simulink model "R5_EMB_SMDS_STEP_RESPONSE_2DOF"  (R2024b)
settings: Solver=ode5  StartTime=0.0  StopTime=S  FixedStep=T  RelTol=1e-3  EnableMultiTasking=on
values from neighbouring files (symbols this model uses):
  Kt = 0.0273    [R5_EMB_SMDS_STEP_RESPONESE_2DOF_script.m]
  r_act = 0.0105    [R5_EMB_SMDS_STEP_RESPONESE_2DOF_script.m]
  T = 0.002    [R5_EMB_SMDS_STEP_RESPONESE_2DOF_script.m]
undefined symbols (not defined in the file or in its folder): Serial_Port, Standard_Devices
libraries: easyio x7, simulink x1

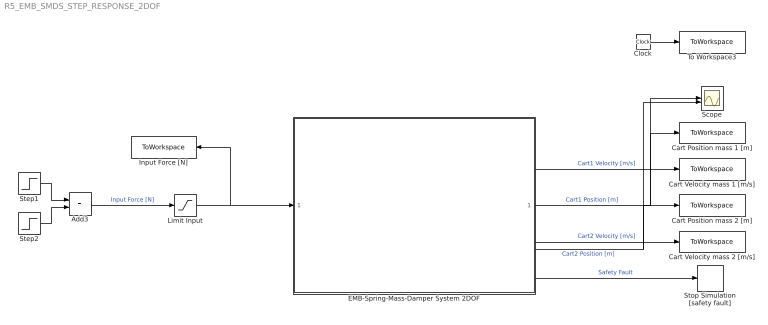
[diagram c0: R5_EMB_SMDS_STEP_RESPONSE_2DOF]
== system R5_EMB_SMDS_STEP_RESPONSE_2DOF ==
  Add3 : Sum
  Cart Position mass 1 [m] : ToWorkspace  VariableName=cart1_position  SampleTime=-1
  Cart Position mass 2 [m] : ToWorkspace  VariableName=cart2_position  SampleTime=-1
  Cart Velocity mass 1 [m/s] : ToWorkspace  VariableName=cart1_velocity  SampleTime=-1
  Cart Velocity mass 2 [m/s] : ToWorkspace  VariableName=cart2_velocity  SampleTime=-1
  Clock : Clock
  EMB-Spring-Mass-Damper System 2DOF : Subsystem
  Input Force [N] : ToWorkspace  VariableName=f_input  SampleTime=-1
  Limit Input : Saturate  UpperLimit=10  LowerLimit=-10
  Scope : Scope  NumInputPorts=2
  Step1 : Step  After=5  SampleTime=0
  Step2 : Step  Time=2  After=-5  SampleTime=0
  Stop Simulation [safety fault] : Stop
  To Workspace3 : ToWorkspace  VariableName=rt_time  SampleTime=-1
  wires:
  Clock/1 -> To Workspace3/1
  EMB-Spring-Mass-Damper System 2DOF/1(Out1) -> Scope/1, Cart Position mass 1 [m]/1  "Cart1 Position [m]"
  EMB-Spring-Mass-Damper System 2DOF/5(Out3) -> Stop Simulation [safety fault]/1  "Safety Fault"
  EMB-Spring-Mass-Damper System 2DOF/2(Out2) -> Cart Velocity mass 1 [m/s]/1  "Cart1 Velocity [m/s]"
  Step1/1 -> Add3/1
  Step2/1 -> Add3/2
  Limit Input/1 -> Input Force [N]/1, EMB-Spring-Mass-Damper System 2DOF/1(In1)
  EMB-Spring-Mass-Damper System 2DOF/3(Out4) -> Scope/2, Cart Position mass 2 [m]/1  "Cart2 Position [m]"
  EMB-Spring-Mass-Damper System 2DOF/4(Out5) -> Cart Velocity mass 2 [m/s]/1  "Cart2 Velocity [m/s]"
  Add3/1 -> Limit Input/1  "Input Force [N]"

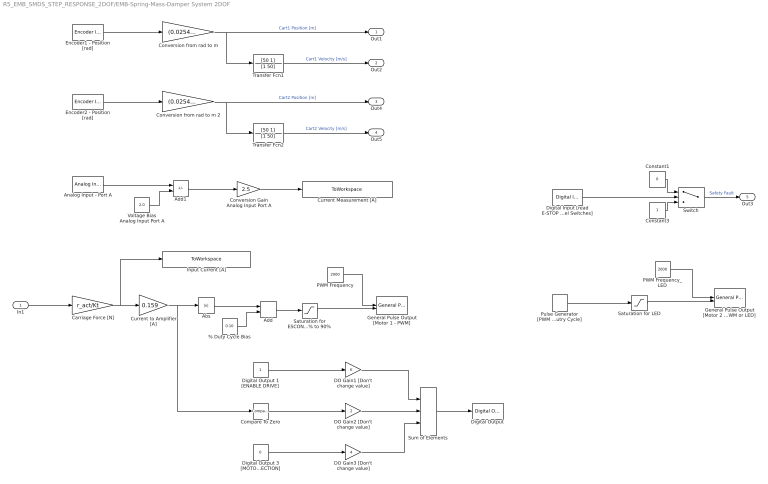
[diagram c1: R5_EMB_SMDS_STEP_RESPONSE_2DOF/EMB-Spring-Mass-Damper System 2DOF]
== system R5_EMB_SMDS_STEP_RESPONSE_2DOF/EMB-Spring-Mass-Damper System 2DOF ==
  In1 : Inport
  % Duty Cycle Bias : Constant  Value=0.10
  Abs : Abs
  Add : Sum
  Add1 : Sum  Inputs=+-
  Analog Input - Port A : easyio/Analog Input  SampleTime=T  MaxMissedTicks=10  ShowMissedTicks=0  YieldWhenWaiting=0  DrvName=Standard_Devices/Serial_Port  DrvAddress=6  DrvOptions=[460800 8 0 0 0 0 0 0]  PacketSize=8  DataTypes='double'  ShowReady=0  ShowError=0  PacketID=1  ByteOrder=1  ShowTimestamp=0  CfgPrm=A6  PrmCfg=unipolar  ResVar=0  VarRes=0
  Carriage Force [N] : Gain  Gain=r_act/Kt
  Compare To Zero : simulink/Logic and Bit Operations/Compare To Zero  relop=>=  OutDataTypeStr=boolean
  Constant1 : Constant  Value=0
  Constant3 : Constant
  Conversion Gain Analog Input Port A : Gain  Gain=2.5
  Conversion from rad to m : Gain  Gain=(0.0254)/(2*pi)
  Conversion from rad to m 2 : Gain  Gain=(0.0254)/(2*pi)
  Current Measurement [A] : ToWorkspace  VariableName=i_measure  SampleTime=-1
  Current to Amplifier [A] : Gain  Gain=0.159
  DO Gain1 [Don't change value] : Gain
  DO Gain2 [Don't change value] : Gain  Gain=2
  DO Gain3 [Don't change value] : Gain  Gain=4
  Digital Input [read E-STOP and End of Travel Switches] : easyio/Digital Input  SampleTime=T  MaxMissedTicks=10  ShowMissedTicks=0  YieldWhenWaiting=0  DrvName=Standard_Devices/Serial_Port  DrvAddress=6  DrvOptions=[460800 8 0 0 0 0 0 0]  PacketSize=8  DataTypes='double'  ShowReady=0  ShowError=0  PacketID=1  ByteOrder=1  ShowTimestamp=0  CfgPrm=D0  PrmCfg=18  ResVar=0  VarRes=0  d7=off  d6=off  d5=off  d4=on  d3=on  d2=off  d1=off  d0=off
  Digital Output : easyio/Digital Output  SampleTime=T  MaxMissedTicks=10  ShowMissedTicks=0  YieldWhenWaiting=0  DrvName=Standard_Devices/Serial_Port  DrvAddress=6  DrvOptions=[460800 8 0 0 0 0 0 0]  PacketSize=8  DataTypes='double'  ShowReady=0  ShowError=0  PacketID=1  ByteOrder=1  InitialValue=0  FinalValue=0  CfgPrm=G0  PrmCfg=F8  ResVar=0  VarRes=0  d7=off  d6=off  d5=off  d4=off  d3=off  d2=on  d1=on  d0=on
  Digital Output 1 [ENABLE DRIVE] : Constant
  Digital Output 3 [MOTOR 2 DIRECTION] : Constant  Value=0
  Encoder1 - Position [rad] : easyio/Encoder Input  SampleTime=T  MaxMissedTicks=10  ShowMissedTicks=0  YieldWhenWaiting=0  DrvName=Standard_Devices/Serial_Port  DrvAddress=6  DrvOptions=[460800 8 0 0 0 0 0 0]  PacketSize=8  DataTypes='double'  ShowReady=0  ShowError=0  PacketID=1  ByteOrder=1  ShowTimestamp=0  CfgPrm=E0  PrmCfg=position  ResVar=0  VarRes=2000
  Encoder2 - Position [rad] : easyio/Encoder Input  SampleTime=T  MaxMissedTicks=10  ShowMissedTicks=0  YieldWhenWaiting=0  DrvName=Standard_Devices/Serial_Port  DrvAddress=6  DrvOptions=[460800 8 0 0 0 0 0 0]  PacketSize=8  DataTypes='double'  ShowReady=0  ShowError=0  PacketID=1  ByteOrder=1  ShowTimestamp=0  CfgPrm=E1  PrmCfg=position  ResVar=0  VarRes=2000
  General Pulse Output [Motor 1 - PWM] : easyio/General Pulse Output  SampleTime=T  MaxMissedTicks=10  ShowMissedTicks=0  YieldWhenWaiting=0  DrvName=Standard_Devices/Serial_Port  DrvAddress=6  DrvOptions=[460800 8 0 0 0 0 0 0]  PacketSize=16  DataTypes={'double','double'}  ShowReady=0  ShowError=0  PacketID=1  ByteOrder=1  InitialValue=[0 0]  FinalValue=[0 0]  CfgPrm=N0  PrmCfg=frequency and duty  ResVar=449.8360 Hz - 115156.25 Hz  VarRes=64
  General Pulse Output [Motor 2 - PWM or LED] : easyio/General Pulse Output  SampleTime=T  MaxMissedTicks=10  ShowMissedTicks=0  YieldWhenWaiting=0  DrvName=Standard_Devices/Serial_Port  DrvAddress=6  DrvOptions=[460800 8 0 0 0 0 0 0]  PacketSize=16  DataTypes={'double','double'}  ShowReady=0  ShowError=0  PacketID=1  ByteOrder=1  InitialValue=[0 0]  FinalValue=[0 0]  CfgPrm=N1  PrmCfg=frequency and duty  ResVar=449.8360 Hz - 115156.25 Hz  VarRes=64
  Input Current [A] : ToWorkspace  VariableName=i_input  SampleTime=-1
  PWM Frequency : Constant  Value=2000
  PWM Frequency_LED : Constant  Value=2000
  Pulse Generator [PWM % Dutry Cycle] : DiscretePulseGenerator  PulseType=Time based  Period=0.4  PulseWidth=50
  Saturation for ESCON 10% to 90% : Saturate  UpperLimit=0.9  LowerLimit=0.1
  Saturation for LED : Saturate  UpperLimit=1  LowerLimit=0
  Sum of Elements : Sum  Inputs=+++
  Switch : Switch  Threshold=8
  Transfer Fcn1 : TransferFcn  Numerator=[50 1]  Denominator=[1 50]
  Transfer Fcn2 : TransferFcn  Numerator=[50 1]  Denominator=[1 50]
  Voltage Bias Analog Input Port A : Constant  Value=2.0
  Out1 : Outport
  Out2 : Outport  Port=2
  Out4 : Outport  Port=3
  Out5 : Outport  Port=4
  Out3 : Outport  Port=5
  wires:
  % Duty Cycle Bias/1 -> Add/2
  Conversion Gain Analog Input Port A/1 -> Current Measurement [A]/1
  Add1/1 -> Conversion Gain Analog Input Port A/1
  Constant1/1 -> Switch/1
  Current to Amplifier [A]/1 -> Abs/1, Compare To Zero/1
  Saturation for ESCON 10% to 90%/1 -> General Pulse Output [Motor 1 - PWM]/2
  Voltage Bias Analog Input Port A/1 -> Add1/2
  DO Gain2 [Don't change value]/1 -> Sum of Elements/2
  Analog Input - Port A/1 -> Add1/1
  PWM Frequency/1 -> General Pulse Output [Motor 1 - PWM]/1
  Conversion from rad to m/1 -> Out1/1, Transfer Fcn1/1  "Cart1 Position [m]"
  DO Gain1 [Don't change value]/1 -> Sum of Elements/1
  Digital Output 1 [ENABLE DRIVE]/1 -> DO Gain1 [Don't change value]/1
  Saturation for LED/1 -> General Pulse Output [Motor 2 - PWM or LED]/2
  Digital Input [read E-STOP and End of Travel Switches]/1 -> Switch/2
  PWM Frequency_LED/1 -> General Pulse Output [Motor 2 - PWM or LED]/1
  Carriage Force [N]/1 -> Input Current [A]/1, Current to Amplifier [A]/1
  Pulse Generator [PWM % Dutry Cycle]/1 -> Saturation for LED/1
  Encoder1 - Position [rad]/1 -> Conversion from rad to m/1
  Sum of Elements/1 -> Digital Output/1
  Add/1 -> Saturation for ESCON 10% to 90%/1
  Constant3/1 -> Switch/3
  Abs/1 -> Add/1
  In1/1 -> Carriage Force [N]/1
  Digital Output 3 [MOTOR 2 DIRECTION]/1 -> DO Gain3 [Don't change value]/1
  DO Gain3 [Don't change value]/1 -> Sum of Elements/3
  Transfer Fcn1/1 -> Out2/1  "Cart1 Velocity [m/s]"
  Conversion from rad to m 2/1 -> Out4/1, Transfer Fcn2/1  "Cart2 Position [m]"
  Encoder2 - Position [rad]/1 -> Conversion from rad to m 2/1
  Transfer Fcn2/1 -> Out5/1  "Cart2 Velocity [m/s]"
  Compare To Zero/1 -> DO Gain2 [Don't change value]/1
  Switch/1 -> Out3/1  "Safety Fault"
